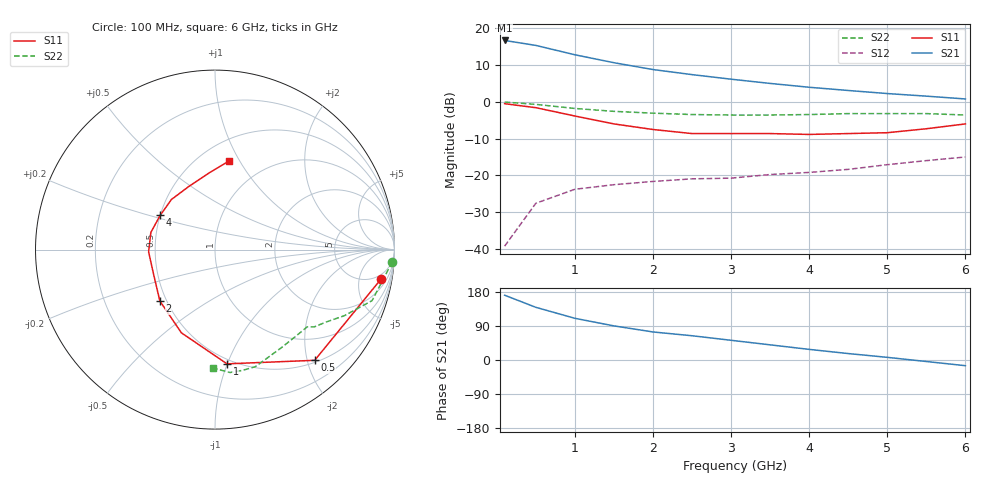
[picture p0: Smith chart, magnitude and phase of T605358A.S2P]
!AT-60535
!S-PARAMETERS at Vce=8V  Ic=2mA.  LAST UPDATED 07-21-92
!OBSOLETED Feb 1994 - nearest replacement: AT-41435
# ghz s ma r 50
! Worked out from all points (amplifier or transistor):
!   13 points, 100 MHz to 6 GHz, reference 50 ohm
!   highest |S21| = 16.6 dB at 100 MHz (marker M1)
!   |S21| within 3 dB of that: start of sweep to 826.3 MHz
!   unconditionally stable (mu >= 1): 2.139 GHz to 5.306 GHz
!   at 1 GHz: K = 0.54, MSG = 18.2 dB, |S12| = -23.7 dB
!   at 3 GHz: K = 1.22, MAG = 10.6 dB, |S12| = -20.7 dB
!   at 6 GHz: K = 0.91, MSG = 7.9 dB, |S12| = -15.0 dB
!   lowest NFmin = 1.40 dB at 1 GHz
!   S11 on the Smith chart (normalised r, x): 100 MHz: 4, -10; 500 MHz: 0.54, -2.13; 1 GHz: 0.46, -1.00; 2 GHz: 0.46, -0.32; 4 GHz: 0.50, +0.22; 6 GHz: 0.69, +0.90
0.1  0.94 -10.0  6.77 171.0  0.011 92.0  0.99 -4.0
0.5  0.83 -48.0  5.8 139.0  0.042 63.0  0.92 -18.0
1  0.64 -84.0  4.33 110.0  0.065 45.0  0.81 -27.0
1.5  0.5 -112.0  3.38 90.0  0.075 41.0  0.74 -33.0
2  0.42 -137.0  2.73 74.0  0.083 37.0  0.7 -38.0
2.5  0.37 -157.0  2.33 64.0  0.09 39.0  0.67 -40.0
3  0.37 -178.0  2.02 52.0  0.092 43.0  0.66 -47.0
3.5  0.37 165.0  1.77 40.0  0.103 41.0  0.66 -56.0
4  0.36 148.0  1.57 28.0  0.11 43.0  0.67 -64.0
4.5  0.37 131.0  1.42 17.0  0.121 43.0  0.69 -71.0
5  0.38 113.0  1.29 7.0  0.14 43.0  0.69 -77.0
5.5  0.43 94.0  1.19 -4.0  0.159 40.0  0.69 -83.0
6  0.5 81.0  1.09 -15.0  0.178 36.0  0.66 -91.0
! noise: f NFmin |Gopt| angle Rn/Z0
1  1.4  0.5  55  0.32
2  1.8  0.4  114  0.38
4  2.8  0.38  -153  0.4
